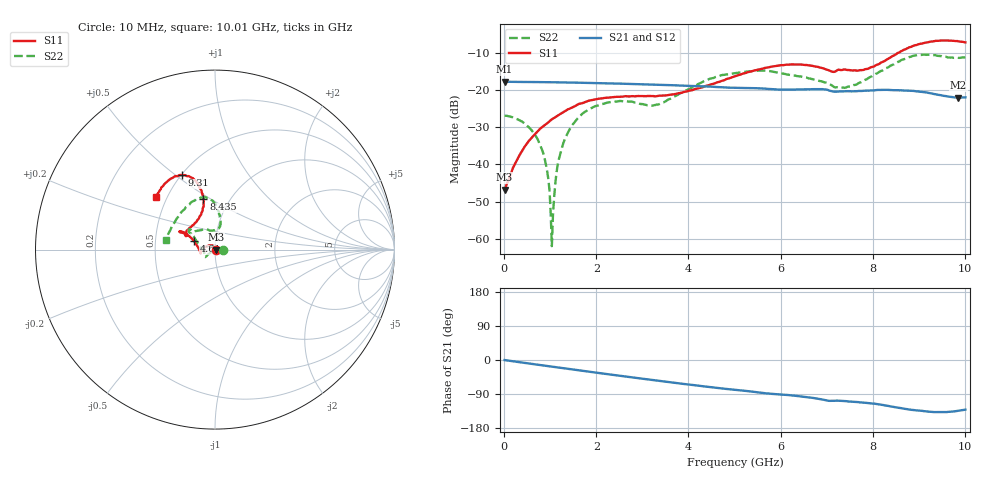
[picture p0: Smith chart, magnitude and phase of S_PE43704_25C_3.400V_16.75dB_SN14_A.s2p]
! Device ID: PE43704
! Dir: z:\PE43704\PE43704_Char_1_20130516\PE43704\AMB\3p400V\16p75dB
! Serial: 14
! Insertion: A
! Impedance: 50 ohm
! Temp: Amb
! VDD: 3.400V
! Attenuation Step: 16.75dB
! IDD: 1.139244e-01mA
#  Hz  S  RI  R  50
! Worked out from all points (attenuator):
!   401 points, 10 MHz to 10.01 GHz, reference 50 ohm
!   highest |S21| = -17.75 dB at 10 MHz (marker M1); lowest = -22.0 dB at 9.86 GHz (marker M2)
!   lowest |S11| = -46.7 dB at 10 MHz (marker M3), VSWR 1.01, Z = 50.5 + j0.0362 ohm
!   |S11| at or under -10 dB: start of sweep to 8.544 GHz
!   |S22| runs from -62.0 to -10.4 dB; largest |S21 - S12| = 0.0014
!   S11 on the Smith chart (normalised r, x): 10 MHz: 1.01, +0.00; 4.61 GHz: 0.79, +0.08; 8.435 GHz: 0.76, +0.46; 9.31 GHz: 0.51, +0.53; 10.01 GHz: 0.44, +0.32
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1e7  0.00459 0.000359  0.1296 -0.00048  0.1297 -0.000423  0.0452 -5.66e-05
3.6e8  -5.63e-05 0.0142  0.1284 -0.014  0.1282 -0.0142  0.0381 0.00526
7.35e8  -0.0155 0.0235  0.1252 -0.0278  0.1252 -0.0277  0.0205 0.00565
9.1e8  -0.0254 0.0238  0.1232 -0.034  0.1232 -0.0339  0.00937 0.00264
9.85e8  -0.0298 0.024  0.1223 -0.0367  0.1223 -0.0366  0.00431 0.00103
1.035e9  -0.0331 0.0233  0.1218 -0.0384  0.1217 -0.0383  0.000335 -0.000721
1.085e9  -0.0358 0.0225  0.1211 -0.0401  0.1211 -0.0401  -0.00277 -0.00233
1.16e9  -0.0402 0.0213  0.1199 -0.0427  0.1199 -0.0427  -0.00843 -0.00497
1.26e9  -0.0457 0.0192  0.1183 -0.0461  0.1183 -0.0461  -0.0151 -0.00832
1.435e9  -0.0551 0.0139  0.1153 -0.0517  0.1152 -0.0516  -0.0261 -0.0161
1.685e9  -0.0663 0.00536  0.1106 -0.0596  0.1106 -0.0595  -0.039 -0.027
2.36e9  -0.0787 -0.0154  0.0952 -0.0777  0.0953 -0.0776  -0.0556 -0.0418
3.36e9  -0.0831 -0.0123  0.0675 -0.0968  0.0676 -0.0967  -0.0642 -0.0061
4.61e9  -0.1171 0.0475  0.031 -0.1058  0.0313 -0.1056  -0.1268 0.0823
5.01e9  -0.1372 0.0689  0.0214 -0.1054  0.0215 -0.1054  -0.1412 0.0929
6.685e9  -0.1898 0.0953  -0.0175 -0.1015  -0.0174 -0.1013  -0.0929 0.1058
7.385e9  -0.1579 0.1051  -0.0304 -0.0913  -0.03 -0.0915  -0.00553 0.1072
8.36e9  -0.0633 0.2621  -0.053 -0.0855  -0.0528 -0.0859  0.0227 0.2066
8.435e9  -0.0641 0.2813  -0.0549 -0.0834  -0.055 -0.084  0.0154 0.2194
9.31e9  -0.1834 0.4138  -0.0657 -0.0605  -0.0656 -0.0604  -0.118 0.2711
9.86e9  -0.3017 0.337  -0.0549 -0.0571  -0.055 -0.0562  -0.2452 0.117
1.001e10  -0.3276 0.2919  -0.0524 -0.0605  -0.0538 -0.0604  -0.2713 0.0558
